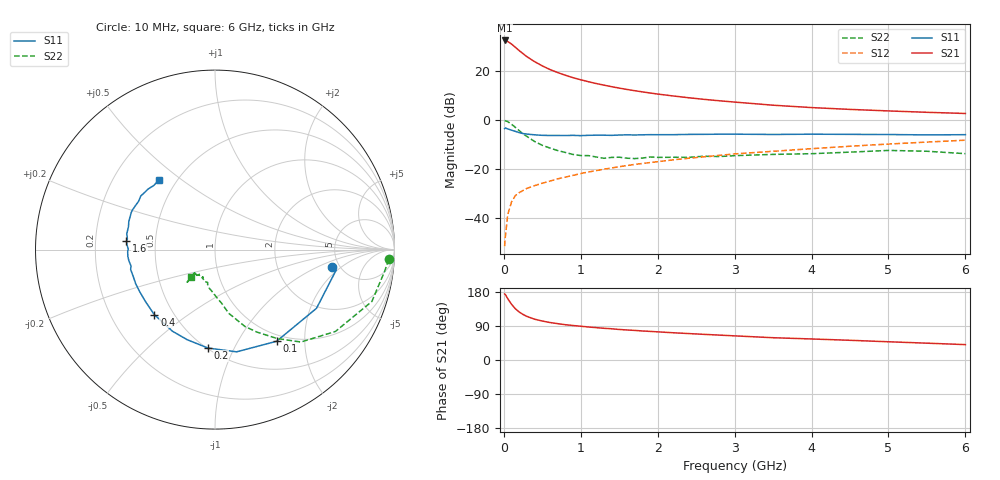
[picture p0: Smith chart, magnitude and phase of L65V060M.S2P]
!  INFINEON TECHNOLOGIES Small Signal Semiconductors
! BFR380L3 , Si-NPN RF-Transistor in TSLP-3-1
!  Vce=5 V,  Ic=60 mA
! Common Emitter S-Parameters:  07. March 2005
#  GHz  S  MA  R  50
! f  S11  S21  S12  S22
! GHz  Mag  Ang  Mag  Ang  Mag  Ang  Mag  Ang
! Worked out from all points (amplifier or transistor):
!   36 points, 10 MHz to 6 GHz, reference 50 ohm
!   highest |S21| = 32.3 dB at 10 MHz (marker M1)
!   |S21| within 3 dB of that: start of sweep to 158.3 MHz
!   unconditionally stable (mu >= 1): 1.587 GHz to 4.802 GHz
!   at 250 MHz: K = 0.47, MSG = 27.8 dB, |S12| = -28.7 dB
!   at 1.4 GHz: K = 0.99, MSG = 16.5 dB, |S12| = -19.6 dB
!   at 6 GHz: K = 0.97, MSG = 5.4 dB, |S12| = -8.3 dB
!   S11 on the Smith chart (normalised r, x): 10 MHz: 4.35, -1.53; 100 MHz: 0.90, -1.48; 200 MHz: 0.51, -0.79; 400 MHz: 0.39, -0.38; 1.6 GHz: 0.34, +0.04; 6 GHz: 0.40, +0.42
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0.01  0.6617 -8.6  41.05 174.4  0.0027 76.0  0.9693 -3.2
0.02  0.6845 -9.6  40.63 172.8  0.0042 90.1  0.9533 -7.2
0.05  0.6534 -30.0  39.14 162.0  0.0117 75.8  0.9205 -18.3
0.1  0.6153 -56.1  34.63 147.0  0.0215 67.3  0.8114 -34.2
0.15  0.5822 -78.1  29.82 135.2  0.0288 59.9  0.703 -47.1
0.2  0.5499 -94.1  25.5 126.5  0.0331 59.1  0.6038 -55.1
0.25  0.5255 -107.1  22.07 120.2  0.0366 55.3  0.516 -63.0
0.3  0.5128 -117.5  19.2 115.0  0.0404 55.3  0.4599 -68.7
0.4  0.4957 -133.0  15.21 107.7  0.046 54.9  0.3625 -77.9
0.5  0.4835 -143.4  12.49 102.8  0.0514 55.9  0.3033 -82.7
0.6  0.4806 -151.0  10.52 98.9  0.0567 58.0  0.2667 -88.0
0.7  0.4812 -156.4  9.133 95.9  0.0631 59.9  0.237 -93.3
0.9  0.4831 -166.7  7.181 91.0  0.0743 62.0  0.1974 -102.1
1.1  0.484 -172.7  5.944 87.1  0.0872 63.6  0.1871 -107.4
1.3  0.4867 -178.6  5.074 83.7  0.0991 64.8  0.1654 -114.1
1.6  0.4954 174.6  4.142 79.2  0.1174 65.6  0.1658 -122.5
2.2  0.4988 165.0  3.055 71.9  0.1533 66.5  0.1733 -125.3
2.8  0.5103 156.2  2.439 65.7  0.1894 66.4  0.1792 -132.1
3.5  0.5037 147.7  1.981 58.8  0.2293 64.4  0.1981 -131.0
4.5  0.5059 141.6  1.628 52.0  0.2902 62.8  0.2203 -130.8
5.5  0.4937 133.6  1.421 44.4  0.3527 59.1  0.2296 -130.3
6  0.4988 128.5  1.345 40.6  0.3854 57.0  0.2051 -131.6
